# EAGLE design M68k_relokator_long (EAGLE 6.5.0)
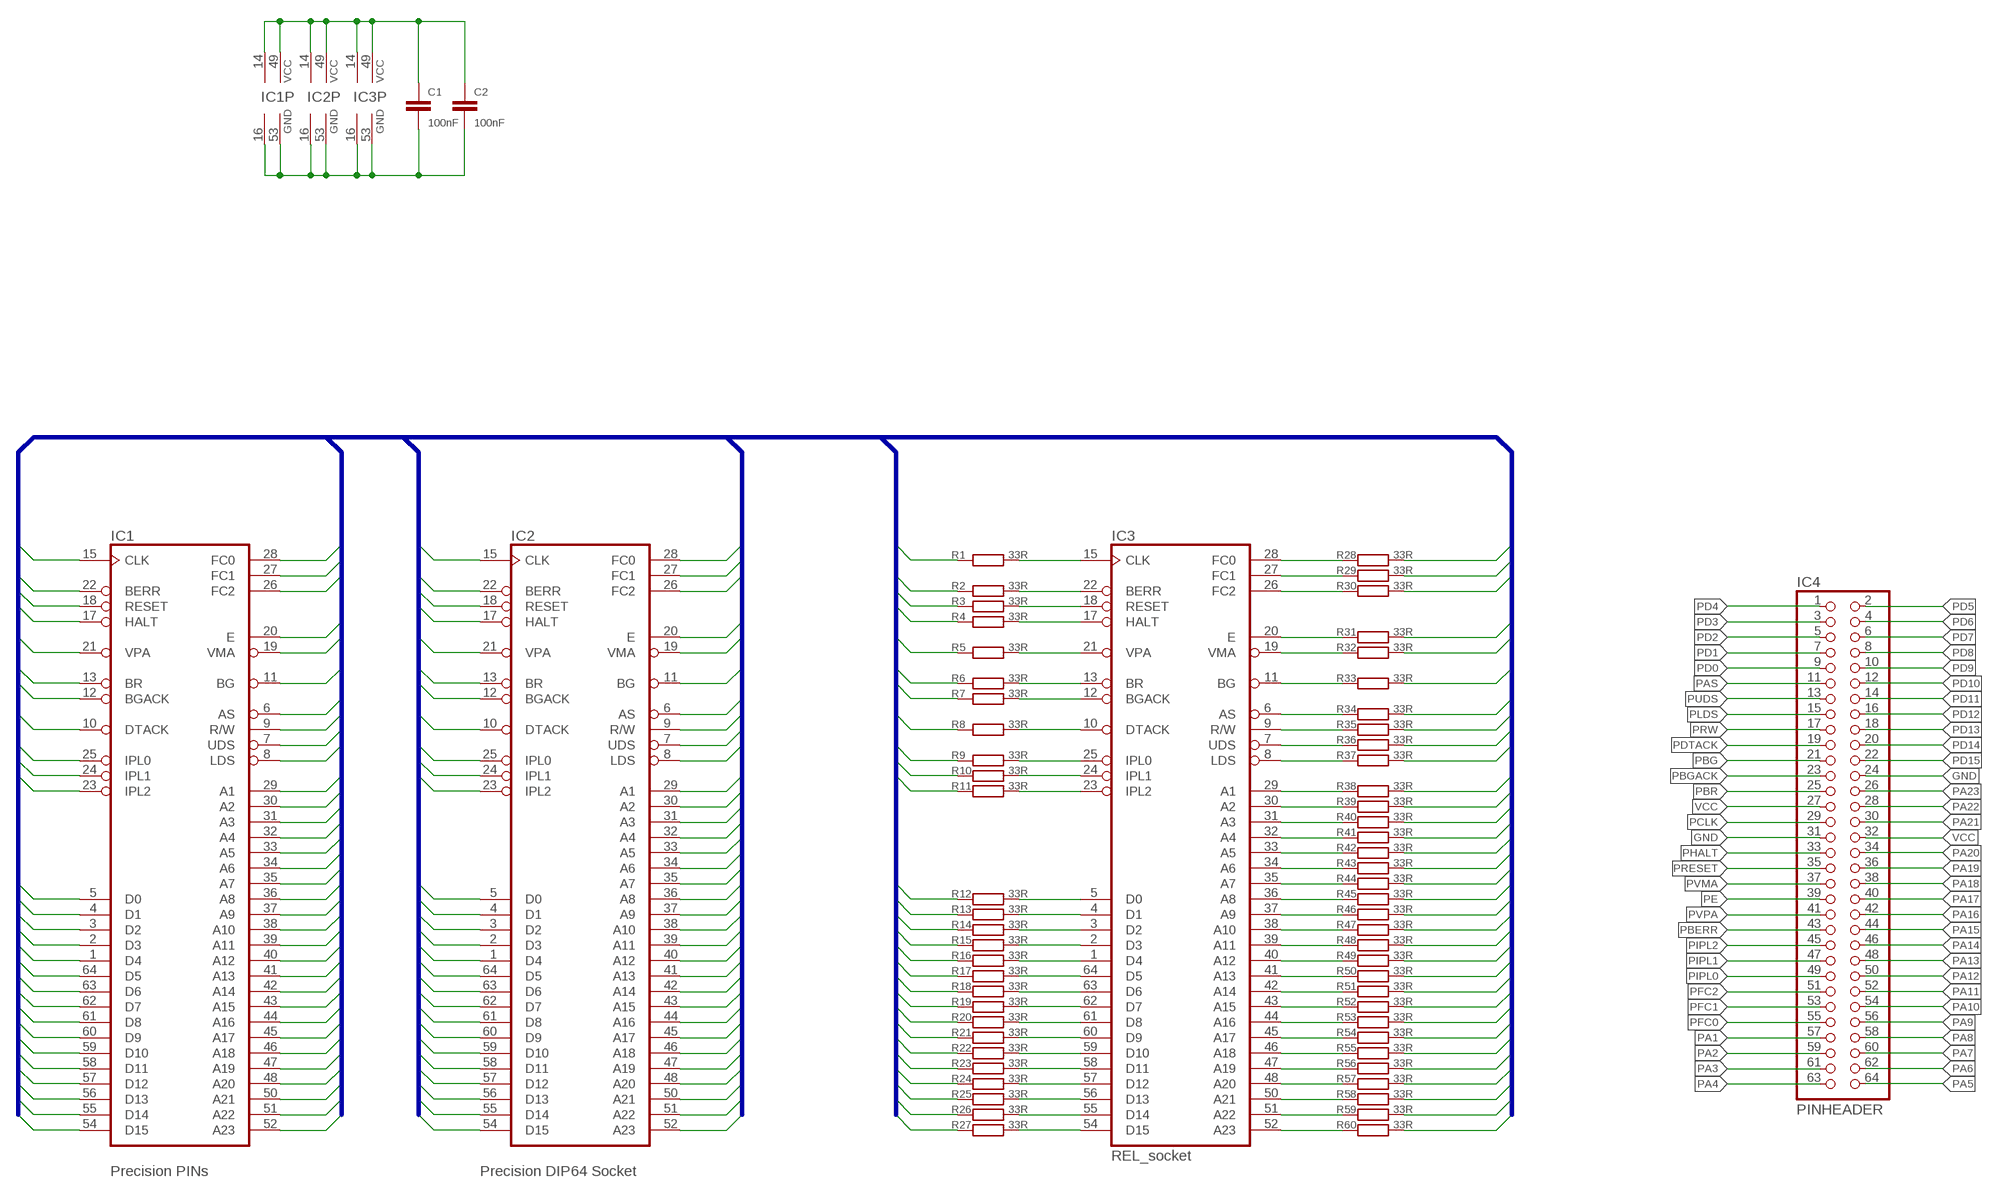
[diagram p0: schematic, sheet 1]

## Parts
C1  100nF  C-EUC0805  [C0805]
C2  100nF  C-EUC0805  [C0805]
IC1  Precision PINs  MC68000P  [DIL64]
IC2  Precision DIP64 Socket  MC68000P  [DIL64]
IC3  REL_socket  MC68000P  [DIL64]
IC4  PINHEADER  PINHD-2X32  [2X32]
R1  33R  R-EU_R0805  [R0805]
R2  33R  R-EU_R0805  [R0805]
R3  33R  R-EU_R0805  [R0805]
R4  33R  R-EU_R0805  [R0805]
R5  33R  R-EU_R0805  [R0805]
R6  33R  R-EU_R0805  [R0805]
R7  33R  R-EU_R0805  [R0805]
R8  33R  R-EU_R0805  [R0805]
R9  33R  R-EU_R0805  [R0805]
R10  33R  R-EU_R0805  [R0805]
R11  33R  R-EU_R0805  [R0805]
R12  33R  R-EU_R0805  [R0805]
R13  33R  R-EU_R0805  [R0805]
R14  33R  R-EU_R0805  [R0805]
R15  33R  R-EU_R0805  [R0805]
R16  33R  R-EU_R0805  [R0805]
R17  33R  R-EU_R0805  [R0805]
R18  33R  R-EU_R0805  [R0805]
R19  33R  R-EU_R0805  [R0805]
R20  33R  R-EU_R0805  [R0805]
R21  33R  R-EU_R0805  [R0805]
R22  33R  R-EU_R0805  [R0805]
R23  33R  R-EU_R0805  [R0805]
R24  33R  R-EU_R0805  [R0805]
R25  33R  R-EU_R0805  [R0805]
R26  33R  R-EU_R0805  [R0805]
R27  33R  R-EU_R0805  [R0805]
R28  33R  R-EU_R0805  [R0805]
R29  33R  R-EU_R0805  [R0805]
R30  33R  R-EU_R0805  [R0805]
R31  33R  R-EU_R0805  [R0805]
R32  33R  R-EU_R0805  [R0805]
R33  33R  R-EU_R0805  [R0805]
R34  33R  R-EU_R0805  [R0805]
R35  33R  R-EU_R0805  [R0805]
R36  33R  R-EU_R0805  [R0805]
R37  33R  R-EU_R0805  [R0805]
R38  33R  R-EU_R0805  [R0805]
R39  33R  R-EU_R0805  [R0805]
R40  33R  R-EU_R0805  [R0805]
R41  33R  R-EU_R0805  [R0805]
R42  33R  R-EU_R0805  [R0805]
R43  33R  R-EU_R0805  [R0805]
R44  33R  R-EU_R0805  [R0805]
R45  33R  R-EU_R0805  [R0805]
R46  33R  R-EU_R0805  [R0805]
R47  33R  R-EU_R0805  [R0805]
R48  33R  R-EU_R0805  [R0805]
R49  33R  R-EU_R0805  [R0805]
R50  33R  R-EU_R0805  [R0805]
R51  33R  R-EU_R0805  [R0805]
R52  33R  R-EU_R0805  [R0805]
R53  33R  R-EU_R0805  [R0805]
R54  33R  R-EU_R0805  [R0805]
R55  33R  R-EU_R0805  [R0805]
R56  33R  R-EU_R0805  [R0805]
R57  33R  R-EU_R0805  [R0805]
R58  33R  R-EU_R0805  [R0805]
R59  33R  R-EU_R0805  [R0805]
R60  33R  R-EU_R0805  [R0805]

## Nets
A1: IC1.29(A1) IC2.29(A1) R38.2
A2: IC1.30(A2) IC2.30(A2) R39.2
A3: IC1.31(A3) IC2.31(A3) R40.2
A4: IC1.32(A4) IC2.32(A4) R41.2
A5: IC1.33(A5) IC2.33(A5) R42.2
A6: IC1.34(A6) IC2.34(A6) R43.2
A7: IC1.35(A7) IC2.35(A7) R44.2
A8: IC1.36(A8) IC2.36(A8) R45.2
A9: IC1.37(A9) IC2.37(A9) R46.2
A10: IC1.38(A10) IC2.38(A10) R47.2
A11: IC1.39(A11) IC2.39(A11) R48.2
A12: IC1.40(A12) IC2.40(A12) R49.2
A13: IC1.41(A13) IC2.41(A13) R50.2
A14: IC1.42(A14) IC2.42(A14) R51.2
A15: IC1.43(A15) IC2.43(A15) R52.2
A16: IC1.44(A16) IC2.44(A16) R53.2
A17: IC1.45(A17) IC2.45(A17) R54.2
A18: IC1.46(A18) IC2.46(A18) R55.2
A19: IC1.47(A19) IC2.47(A19) R56.2
A20: IC1.48(A20) IC2.48(A20) R57.2
A21: IC1.50(A21) IC2.50(A21) R58.2
A22: IC1.51(A22) IC2.51(A22) R59.2
A23: IC1.52(A23) IC2.52(A23) R60.2
AS: IC1.6(AS) IC2.6(AS) R34.2
BERR: IC1.22(BERR) IC2.22(BERR) R2.1
BG: IC1.11(BG) IC2.11(BG) R33.2
BGACK: IC1.12(BGACK) IC2.12(BGACK) R7.1
BR: IC1.13(BR) IC2.13(BR) R6.1
CLK: IC1.15(CLK) IC2.15(CLK) R1.1
D0: IC1.5(D0) IC2.5(D0) R12.1
D1: IC1.4(D1) IC2.4(D1) R13.1
D2: IC1.3(D2) IC2.3(D2) R14.1
D3: IC1.2(D3) IC2.2(D3) R15.1
D4: IC1.1(D4) IC2.1(D4) R16.1
D5: IC1.64(D5) IC2.64(D5) R17.1
D6: IC1.63(D6) IC2.63(D6) R18.1
D7: IC1.62(D7) IC2.62(D7) R19.1
D8: IC1.61(D8) IC2.61(D8) R20.1
D9: IC1.60(D9) IC2.60(D9) R21.1
D10: IC1.59(D10) IC2.59(D10) R22.1
D11: IC1.58(D11) IC2.58(D11) R23.1
D12: IC1.57(D12) IC2.57(D12) R24.1
D13: IC1.56(D13) IC2.56(D13) R25.1
D14: IC1.55(D14) IC2.55(D14) R26.1
D15: IC1.54(D15) IC2.54(D15) R27.1
DTACK: IC1.10(DTACK) IC2.10(DTACK) R8.1
E: IC1.20(E) IC2.20(E) R31.2
FC0: IC1.28(FC0) IC2.28(FC0) R28.2
FC1: IC1.27(FC1) IC2.27(FC1) R29.2
FC2: IC1.26(FC2) IC2.26(FC2) R30.2
GND: C1.2 C2.2 IC1.16(GND) IC1.53(GND) IC2.16(GND) IC2.53(GND) IC3.16(GND) IC3.53(GND) IC4.24 IC4.31
HALT: IC1.17(HALT) IC2.17(HALT) R4.1
IPL0: IC1.25(IPL0) IC2.25(IPL0) R9.1
IPL1: IC1.24(IPL1) IC2.24(IPL1) R10.1
IPL2: IC1.23(IPL2) IC2.23(IPL2) R11.1
LDS: IC1.8(LDS) IC2.8(LDS) R37.2
PA1: IC3.29(A1) IC4.57 R38.1
PA2: IC3.30(A2) IC4.59 R39.1
PA3: IC3.31(A3) IC4.61 R40.1
PA4: IC3.32(A4) IC4.63 R41.1
PA5: IC3.33(A5) IC4.64 R42.1
PA6: IC3.34(A6) IC4.62 R43.1
PA7: IC3.35(A7) IC4.60 R44.1
PA8: IC3.36(A8) IC4.58 R45.1
PA9: IC3.37(A9) IC4.56 R46.1
PA10: IC3.38(A10) IC4.54 R47.1
PA11: IC3.39(A11) IC4.52 R48.1
PA12: IC3.40(A12) IC4.50 R49.1
PA13: IC3.41(A13) IC4.48 R50.1
PA14: IC3.42(A14) IC4.46 R51.1
PA15: IC3.43(A15) IC4.44 R52.1
PA16: IC3.44(A16) IC4.42 R53.1
PA17: IC3.45(A17) IC4.40 R54.1
PA18: IC3.46(A18) IC4.38 R55.1
PA19: IC3.47(A19) IC4.36 R56.1
PA20: IC3.48(A20) IC4.34 R57.1
PA21: IC3.50(A21) IC4.30 R58.1
PA22: IC3.51(A22) IC4.28 R59.1
PA23: IC3.52(A23) IC4.26 R60.1
PAS: IC3.6(AS) IC4.11 R34.1
PBERR: IC3.22(BERR) IC4.43 R2.2
PBG: IC3.11(BG) IC4.21 R33.1
PBGACK: IC3.12(BGACK) IC4.23 R7.2
PBR: IC3.13(BR) IC4.25 R6.2
PCLK: IC3.15(CLK) IC4.29 R1.2
PD0: IC3.5(D0) IC4.9 R12.2
PD1: IC3.4(D1) IC4.7 R13.2
PD2: IC3.3(D2) IC4.5 R14.2
PD3: IC3.2(D3) IC4.3 R15.2
PD4: IC3.1(D4) IC4.1 R16.2
PD5: IC3.64(D5) IC4.2 R17.2
PD6: IC3.63(D6) IC4.4 R18.2
PD7: IC3.62(D7) IC4.6 R19.2
PD8: IC3.61(D8) IC4.8 R20.2
PD9: IC3.60(D9) IC4.10 R21.2
PD10: IC3.59(D10) IC4.12 R22.2
PD11: IC3.58(D11) IC4.14 R23.2
PD12: IC3.57(D12) IC4.16 R24.2
PD13: IC3.56(D13) IC4.18 R25.2
PD14: IC3.55(D14) IC4.20 R26.2
PD15: IC3.54(D15) IC4.22 R27.2
PDTACK: IC3.10(DTACK) IC4.19 R8.2
PE: IC3.20(E) IC4.39 R31.1
PFC0: IC3.28(FC0) IC4.55 R28.1
PFC1: IC3.27(FC1) IC4.53 R29.1
PFC2: IC3.26(FC2) IC4.51 R30.1
PHALT: IC3.17(HALT) IC4.33 R4.2
PIPL0: IC3.25(IPL0) IC4.49 R9.2
PIPL1: IC3.24(IPL1) IC4.47 R10.2
PIPL2: IC3.23(IPL2) IC4.45 R11.2
PLDS: IC3.8(LDS) IC4.15 R37.1
PRESET: IC3.18(RESET) IC4.35 R3.2
PRW: IC3.9(R/W) IC4.17 R35.1
PUDS: IC3.7(UDS) IC4.13 R36.1
PVMA: IC3.19(VMA) IC4.37 R32.1
PVPA: IC3.21(VPA) IC4.41 R5.2
RESET: IC1.18(RESET) IC2.18(RESET) R3.1
RW: IC1.9(R/W) IC2.9(R/W) R35.2
UDS: IC1.7(UDS) IC2.7(UDS) R36.2
VCC: C1.1 C2.1 IC1.14(VCC) IC1.49(VCC) IC2.14(VCC) IC2.49(VCC) IC3.14(VCC) IC3.49(VCC) IC4.27 IC4.32
VMA: IC1.19(VMA) IC2.19(VMA) R32.2
VPA: IC1.21(VPA) IC2.21(VPA) R5.1

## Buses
D[0..15],IPL[0..2],DTACK,BGACK,BR,VPA,HALT,RESET,BERR,CLK,FC[0..2],E,VMA,BG,AS,RW,UDS,LDS,A[1..23]

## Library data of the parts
C1 C2 = rcl:C-EU: CAPACITOR, European symbol
IC1-IC3 = micro-mc68000:MC68000P: 68xxx PROCESSOR; OC_FARNELL: unknown; OC_NEWARK: unknown
IC4 = pinhead:PINHD-2X32
R1-R60 = rcl:R-EU_: RESISTOR, European symbol

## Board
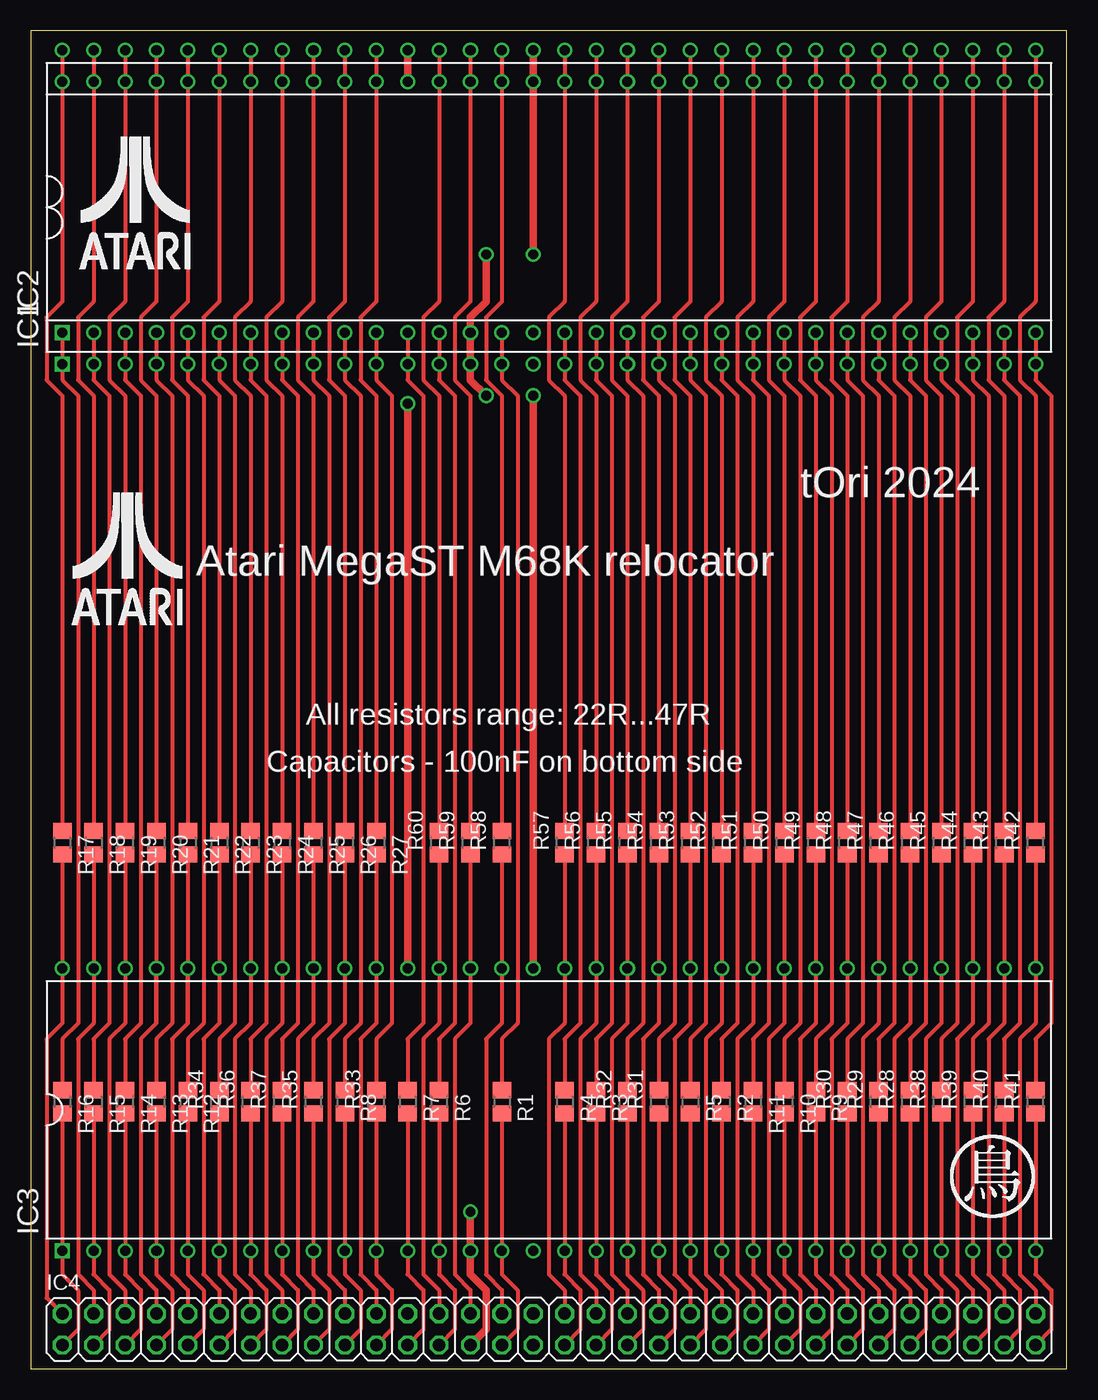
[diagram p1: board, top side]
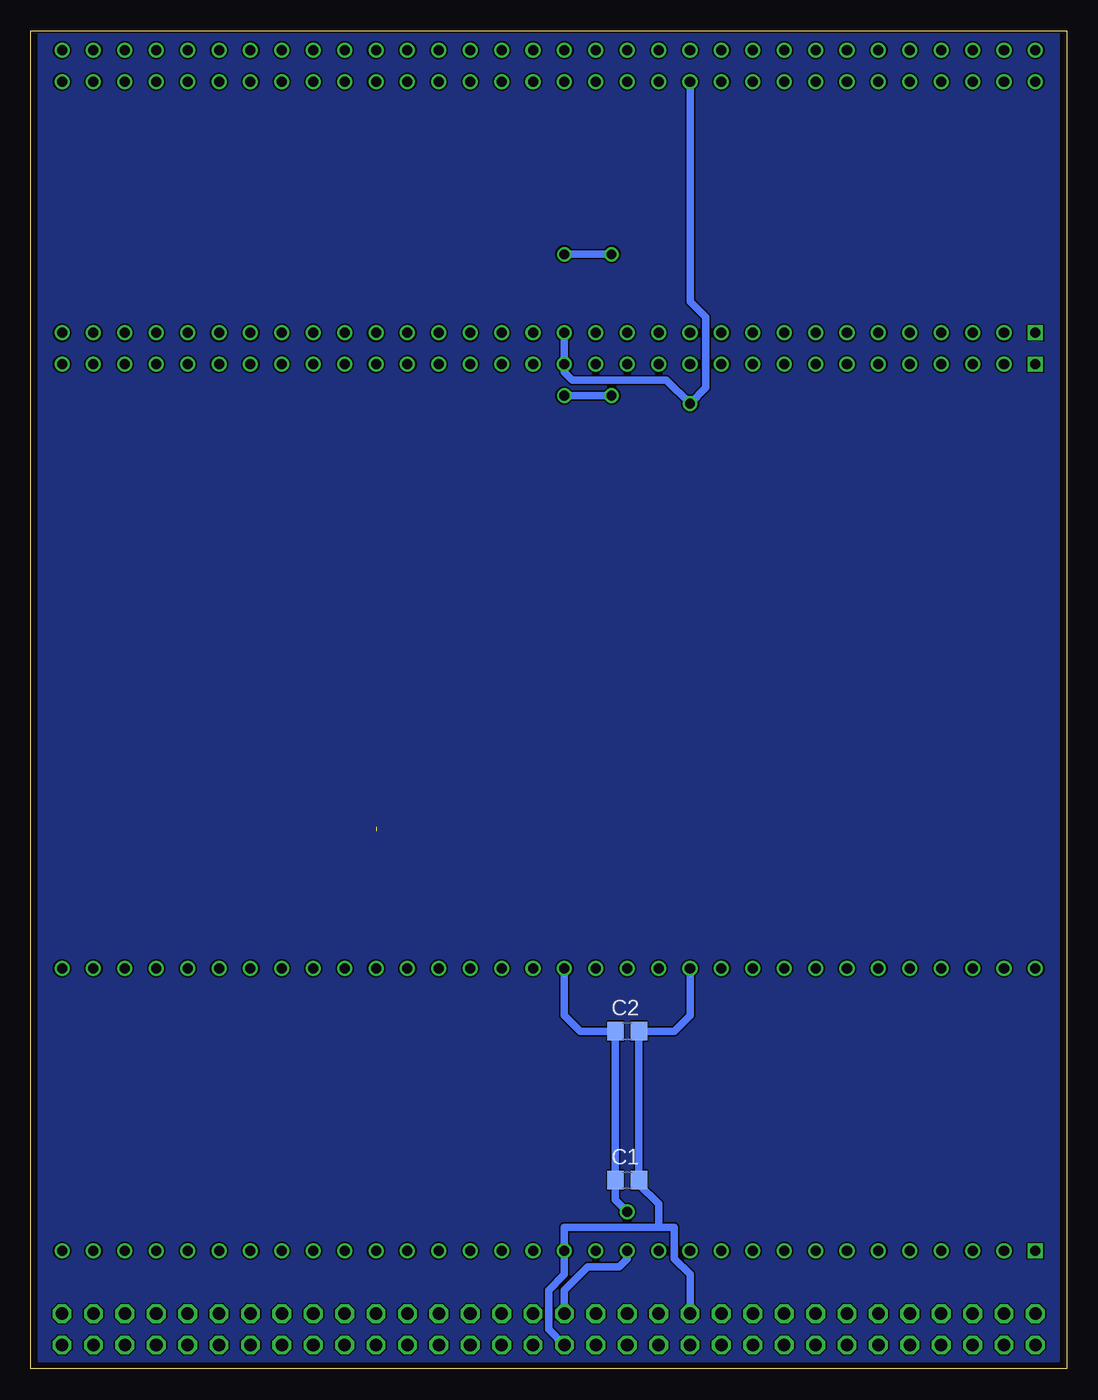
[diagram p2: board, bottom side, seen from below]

Size 83.8 x 108.26 mm. Coordinates in mm from the lower left corner, seen from the top.
Outline: 0,0 83.8,0 83.8,108.26 0,108.26 0,0
Copper layers (1*16): Top 0.035mm / dielectric 0.2mm / Bottom 0.035mm
Design rules "jlcpcb-2-layer": minimum track width 3.5mil, minimum drill 0.2mm, track to track 5mil, track to pad 5mil, pad to pad 5mil, via to via 5mil, smd to smd 0mil, copper to edge 0.1mm, drill to drill 5mil, minimum pad ring 4mil, minimum via ring 4mil, stop-mask expansion 3mil, vias tented up to drill 100mil, thermal gap 10mil

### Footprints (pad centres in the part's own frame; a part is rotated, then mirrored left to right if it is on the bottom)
C0805 = smd 1.3 x 1.5: 1 -0.95,0; 2 0.95,0
DIL64 = drill 0.813 square: 1 -39.37,-11.43 | drill 0.813: 2 -36.83,-11.43; 3 -34.29,-11.43; 4 -31.75,-11.43; 5 -29.21,-11.43; 6 -26.67,-11.43; 7 -24.13,-11.43; 8 -21.59,-11.43; 9 -19.05,-11.43; 10 -16.51,-11.43; 11 -13.97,-11.43; 12 -11.43,-11.43; 13 -8.89,-11.43; 14 -6.35,-11.43; 15 -3.81,-11.43; 16 -1.27,-11.43; 17 1.27,-11.43; 18 3.81,-11.43; 19 6.35,-11.43; 20 8.89,-11.43; 21 11.43,-11.43; 22 13.97,-11.43; 23 16.51,-11.43; 24 19.05,-11.43; 25 21.59,-11.43; 26 24.13,-11.43; 27 26.67,-11.43; 28 29.21,-11.43; 29 31.75,-11.43; 30 34.29,-11.43; 31 36.83,-11.43; 32 39.37,-11.43; 33 39.37,11.43; 34 36.83,11.43; 35 34.29,11.43; 36 31.75,11.43; 37 29.21,11.43; 38 26.67,11.43; 39 24.13,11.43; 40 21.59,11.43; 41 19.05,11.43; 42 16.51,11.43; 43 13.97,11.43; 44 11.43,11.43; 45 8.89,11.43; 46 6.35,11.43; 47 3.81,11.43; 48 1.27,11.43; 49 -1.27,11.43; 50 -3.81,11.43; 51 -6.35,11.43; 52 -8.89,11.43; 53 -11.43,11.43; 54 -13.97,11.43; 55 -16.51,11.43; 56 -19.05,11.43; 57 -21.59,11.43; 58 -24.13,11.43; 59 -26.67,11.43; 60 -29.21,11.43; 61 -31.75,11.43; 62 -34.29,11.43; 63 -36.83,11.43; 64 -39.37,11.43
2X32 = drill 1.016 octagon: 1 -36.83,-1.27; 2 -36.83,1.27; 3 -34.29,-1.27; 4 -34.29,1.27; 5 -31.75,-1.27; 6 -31.75,1.27; 7 -29.21,-1.27; 8 -29.21,1.27; 9 -26.67,-1.27; 10 -26.67,1.27; 11 -24.13,-1.27; 12 -24.13,1.27; 13 -21.59,-1.27; 14 -21.59,1.27; 15 -19.05,-1.27; 16 -19.05,1.27; 17 -16.51,-1.27; 18 -16.51,1.27; 19 -13.97,-1.27; 20 -13.97,1.27; 21 -11.43,-1.27; 22 -11.43,1.27; 23 -8.89,-1.27; 24 -8.89,1.27; 25 -6.35,-1.27; 26 -6.35,1.27; 27 -3.81,-1.27; 28 -3.81,1.27; 29 -1.27,-1.27; 30 -1.27,1.27; 31 1.27,-1.27; 32 1.27,1.27; 33 3.81,-1.27; 34 3.81,1.27; 35 6.35,-1.27; 36 6.35,1.27; 37 8.89,-1.27; 38 8.89,1.27; 39 11.43,-1.27; 40 11.43,1.27; 41 13.97,-1.27; 42 13.97,1.27; 43 16.51,-1.27; 44 16.51,1.27; 45 19.05,-1.27; 46 19.05,1.27; 47 21.59,-1.27; 48 21.59,1.27; 49 24.13,-1.27; 50 24.13,1.27; 51 26.67,-1.27; 52 26.67,1.27; 53 29.21,-1.27; 54 29.21,1.27; 55 31.75,-1.27; 56 31.75,1.27; 57 34.29,-1.27; 58 34.29,1.27; 59 36.83,-1.27; 60 36.83,1.27; 61 39.37,-1.27; 62 39.37,1.27; 63 41.91,-1.27; 64 41.91,1.27
R0805 = smd 1.3 x 1.5: 1 -0.95,0; 2 0.95,0

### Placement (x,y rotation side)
C1  35.56,15.24 0 bottom
C2  35.56,27.31 0 bottom
IC1  41.91,92.71 0 top
IC2  41.91,95.25 0 top
IC3  41.91,20.96 0 top
IC4  39.37,3.18 0 top
R1  38.1,21.59 270 top
R2  55.88,21.59 270 top
R3  45.72,21.59 270 top
R4  43.18,21.59 270 top
R5  53.34,21.59 270 top
R6  33.02,21.59 270 top
R7  30.48,21.59 270 top
R8  25.4,21.59 270 top
R9  63.5,21.59 270 top
R10  60.96,21.59 270 top
R11  58.42,21.59 270 top
R12  12.7,21.59 270 top
R13  10.16,21.59 270 top
R14  7.62,21.59 270 top
R15  5.08,21.59 270 top
R16  2.54,21.59 270 top
R17  2.54,42.55 270 top
R18  5.08,42.55 270 top
R19  7.62,42.55 270 top
R20  10.16,42.55 270 top
R21  12.7,42.55 270 top
R22  15.24,42.55 270 top
R23  17.78,42.55 270 top
R24  20.32,42.55 270 top
R25  22.86,42.55 270 top
R26  25.4,42.55 270 top
R27  27.94,42.55 270 top
R28  71.12,21.59 90 top
R29  68.58,21.59 90 top
R30  66.04,21.59 90 top
R31  50.8,21.59 90 top
R32  48.26,21.59 90 top
R33  27.94,21.59 90 top
R34  15.24,21.59 90 top
R35  22.86,21.59 90 top
R36  17.78,21.59 90 top
R37  20.32,21.59 90 top
R38  73.66,21.59 90 top
R39  76.2,21.59 90 top
R40  78.74,21.59 90 top
R41  81.28,21.59 90 top
R42  81.28,42.55 90 top
R43  78.74,42.55 90 top
R44  76.2,42.55 90 top
R45  73.66,42.55 90 top
R46  71.12,42.55 90 top
R47  68.58,42.55 90 top
R48  66.04,42.55 90 top
R49  63.5,42.55 90 top
R50  60.96,42.55 90 top
R51  58.42,42.55 90 top
R52  55.88,42.55 90 top
R53  53.34,42.55 90 top
R54  50.8,42.55 90 top
R55  48.26,42.55 90 top
R56  45.72,42.55 90 top
R57  43.18,42.55 90 top
R58  38.1,42.55 90 top
R59  35.56,42.55 90 top
R60  33.02,42.55 90 top

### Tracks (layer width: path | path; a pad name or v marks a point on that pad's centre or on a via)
A1
  Top 0.305: IC2.29 IC1.29 73.66,80.01 74.93,78.74 74.93,27.94 73.66,26.67 R38.2
A2
  Top 0.305: IC2.30 IC1.30 76.2,80.01 77.47,78.74 77.47,27.94 76.2,26.67 R39.2
A3
  Top 0.305: IC2.31 IC1.31 78.74,80.01 80.01,78.74 80.01,27.94 78.74,26.67 R40.2
A4
  Top 0.305: IC2.32 IC1.32 81.28,80.01 82.55,78.74 82.55,27.94 81.28,26.67 R41.2
A5
  Top 0.305: IC2.33 IC1.33 81.28,86.36 80.01,85.09 80.01,80.01 81.28,78.74 R42.2
A6
  Top 0.305: IC2.34 IC1.34 78.74,86.36 77.47,85.09 77.47,80.01 78.74,78.74 R43.2
A7
  Top 0.305: IC2.35 IC1.35 76.2,86.36 74.93,85.09 74.93,80.01 76.2,78.74 R44.2
A8
  Top 0.305: IC2.36 IC1.36 73.66,86.36 72.39,85.09 72.39,80.01 73.66,78.74 R45.2
A9
  Top 0.305: IC2.37 IC1.37 71.12,86.36 69.85,85.09 69.85,80.01 71.12,78.74 R46.2
A10
  Top 0.305: IC2.38 IC1.38 68.58,86.36 67.31,85.09 67.31,80.01 68.58,78.74 R47.2
A11
  Top 0.305: IC2.39 IC1.39 66.04,86.36 64.77,85.09 64.77,80.01 66.04,78.74 R48.2
A12
  Top 0.305: IC2.40 IC1.40 63.5,86.36 62.23,85.09 62.23,80.01 63.5,78.74 R49.2
A13
  Top 0.305: IC2.41 IC1.41 60.96,86.36 59.69,85.09 59.69,80.01 60.96,78.74 R50.2
A14
  Top 0.305: IC2.42 IC1.42 58.42,86.36 57.15,85.09 57.15,80.01 58.42,78.74 R51.2
A15  (1 unrouted)
  Top 0.305: IC2.43 IC1.43 55.88,86.36 54.61,85.09 54.61,80.01 55.88,78.74 55.88,43.82
A16
  Top 0.305: IC2.44 IC1.44 53.34,86.36 52.07,85.09 52.07,80.01 53.34,78.74 R53.2
A17
  Top 0.305: IC2.45 IC1.45 50.8,86.36 49.53,85.09 49.53,80.01 50.8,78.74 R54.2
A18
  Top 0.305: IC2.46 IC1.46 48.26,86.36 46.99,85.09 46.99,80.01 48.26,78.74 R55.2
A19
  Top 0.305: IC2.47 IC1.47 45.72,86.36 44.45,85.09 44.45,80.01 45.72,78.74 R56.2
A20
  Top 0.305: IC2.48 IC1.48 43.18,86.36 41.91,85.09 41.91,80.01 43.18,78.74 R57.2
A21
  Top 0.305: IC2.50 IC1.50 38.1,86.36 36.83,85.09 36.83,80.01 38.1,78.74 R58.2
A22
  Top 0.305: IC2.51 IC1.51 35.56,86.36 34.29,85.09 34.29,80.01 35.56,78.74 R59.2
A23
  Top 0.305: IC2.52 IC1.52 33.02,86.36 31.75,85.09 31.75,80.01 33.02,78.74 R60.2
AS
  Top 0.305: IC2.6 IC1.6 15.24,80.01 16.51,78.74 16.51,27.94 15.24,26.67 R34.2
BERR
  Top 0.305: IC2.22 IC1.22 55.88,80.01 57.15,78.74 57.15,27.94 55.88,26.67 R2.1
BG
  Top 0.305: IC2.11 IC1.11 27.94,80.01 29.21,78.74 29.21,27.94 27.94,26.67 R33.2
BGACK
  Top 0.305: IC2.12 IC1.12 30.48,80.01 31.75,78.74 31.75,27.94 30.48,26.67 R7.1
BR
  Top 0.305: IC2.13 IC1.13 33.02,80.01 34.29,78.74 34.29,27.94 33.02,26.67 R6.1
CLK
  Top 0.305: IC2.15 IC1.15 38.1,80.01 39.37,78.74 39.37,27.94 38.1,26.67 R1.1
D0
  Top 0.305: IC2.5 IC1.5 12.7,80.01 13.97,78.74 13.97,27.94 12.7,26.67 R12.1
D1
  Top 0.305: IC2.4 IC1.4 10.16,80.01 11.43,78.74 11.43,27.94 10.16,26.67 R13.1
D2
  Top 0.305: IC2.3 IC1.3 7.62,80.01 8.89,78.74 8.89,27.94 7.62,26.67 R14.1
D3
  Top 0.305: IC2.2 IC1.2 5.08,80.01 6.35,78.74 6.35,27.94 5.08,26.67 R15.1
D4
  Top 0.305: IC2.1 IC1.1 2.54,80.01 3.81,78.74 3.81,27.94 2.54,26.67 R16.1
D5
  Top 0.305: IC2.64 IC1.64 2.54,86.36 1.27,85.09 1.27,80.01 2.54,78.74 R17.1
D6
  Top 0.305: IC2.63 IC1.63 5.08,86.36 3.81,85.09 3.81,80.01 5.08,78.74 R18.1
D7
  Top 0.305: IC2.62 IC1.62 7.62,86.36 6.35,85.09 6.35,80.01 7.62,78.74 R19.1
D8
  Top 0.305: IC2.61 IC1.61 10.16,86.36 8.89,85.09 8.89,80.01 10.16,78.74 R20.1
D9
  Top 0.305: IC2.60 IC1.60 12.7,86.36 11.43,85.09 11.43,80.01 12.7,78.74 R21.1
D10
  Top 0.305: IC2.59 IC1.59 15.24,86.36 13.97,85.09 13.97,80.01 15.24,78.74 R22.1
D11
  Top 0.305: IC2.58 IC1.58 17.78,86.36 16.51,85.09 16.51,80.01 17.78,78.74 R23.1
D12
  Top 0.305: IC2.57 IC1.57 20.32,86.36 19.05,85.09 19.05,80.01 20.32,78.74 R24.1
D13
  Top 0.305: IC2.56 IC1.56 22.86,86.36 21.59,85.09 21.59,80.01 22.86,78.74 R25.1
D14
  Top 0.305: IC2.55 IC1.55 25.4,86.36 24.13,85.09 24.13,80.01 25.4,78.74 R26.1
D15
  Top 0.305: IC2.54 IC1.54 27.94,86.36 26.67,85.09 26.67,80.01 27.94,78.74 R27.1
DTACK
  Top 0.305: IC2.10 IC1.10 25.4,80.01 26.67,78.74 26.67,27.94 25.4,26.67 R8.1
E
  Top 0.305: IC2.20 IC1.20 50.8,80.01 52.07,78.74 52.07,27.94 50.8,26.67 R31.2
FC0
  Top 0.305: IC2.28 IC1.28 71.12,80.01 72.39,78.74 72.39,27.94 71.12,26.67 R28.2
FC1
  Top 0.305: IC2.27 IC1.27 68.58,80.01 69.85,78.74 69.85,27.94 68.58,26.67 R29.2
FC2
  Top 0.305: IC2.26 IC1.26 66.04,80.01 67.31,78.74 67.31,27.94 66.04,26.67 R30.2
GND  (via drill 0.8)
  Top 0.61: IC2.53 IC1.53 | v30.48,78.11 IC3.53
  Bottom 0.61: IC3.53 30.48,28.58 31.75,27.31 C2.2 C1.2 34.61,14.93 33.02,13.34 33.02,11.43 | 33.02,11.43 40.64,11.43 IC3.16 40.64,7.62 41.91,6.35 41.91,3.18 IC4.31 | IC4.24 30.48,7.62 31.75,8.89 31.75,11.43 33.02,11.43 | IC2.16 IC1.16 40.64,80.65 40.01,80.01 32.38,80.01 v30.48,78.11 29.21,79.38 29.21,85.09 30.48,86.36 IC1.53
HALT
  Top 0.305: IC2.17 IC1.17 43.18,80.01 44.45,78.74 44.45,27.94 43.18,26.67 R4.1
IPL0
  Top 0.305: IC2.25 IC1.25 63.5,80.01 64.77,78.74 64.77,27.94 63.5,26.67 R9.1
IPL1
  Top 0.305: IC2.24 IC1.24 60.96,80.01 62.23,78.74 62.23,27.94 60.96,26.67 R10.1
IPL2
  Top 0.305: IC2.23 IC1.23 58.42,80.01 59.69,78.74 59.69,27.94 58.42,26.67 R11.1
LDS
  Top 0.305: IC2.8 IC1.8 20.32,80.01 21.59,78.74 21.59,27.94 20.32,26.67 R37.2
N$1
  pour Bottom: 0.64,107.95 83.19,107.95 83.19,0.64 0.64,0.64
PA1
  Top 0.305: R38.1 IC3.29 73.66,7.62 74.93,6.35 74.93,3.18 IC4.57
PA2
  Top 0.305: R39.1 IC3.30 76.2,7.62 77.47,6.35 77.47,3.18 IC4.59
PA3
  Top 0.305: R40.1 IC3.31 78.74,7.62 80.01,6.35 80.01,3.18 IC4.61
PA4
  Top 0.305: R41.1 IC3.32 81.28,7.62 82.55,6.35 82.55,3.18 IC4.63
PA5
  Top 0.305: R42.1 IC3.33 81.28,27.94 80.01,26.67 80.01,7.62 81.28,6.35 IC4.64
PA6
  Top 0.305: R43.1 IC3.34 78.74,27.94 77.47,26.67 77.47,7.62 78.74,6.35 IC4.62
PA7
  Top 0.305: R44.1 IC3.35 76.2,27.94 74.93,26.67 74.93,7.62 76.2,6.35 IC4.60
PA8
  Top 0.305: R45.1 IC3.36 73.66,27.94 72.39,26.67 72.39,7.62 73.66,6.35 IC4.58
PA9
  Top 0.305: R46.1 IC3.37 71.12,27.94 69.85,26.67 69.85,7.62 71.12,6.35 IC4.56
PA10
  Top 0.305: R47.1 IC3.38 68.58,27.94 67.31,26.67 67.31,7.62 68.58,6.35 IC4.54
PA11
  Top 0.305: R48.1 IC3.39 66.04,27.94 64.77,26.67 64.77,7.62 66.04,6.35 IC4.52
PA12
  Top 0.305: R49.1 IC3.40 63.5,27.94 62.23,26.67 62.23,7.62 63.5,6.35 IC4.50
PA13
  Top 0.305: R50.1 IC3.41 60.96,27.94 59.69,26.67 59.69,7.62 60.96,6.35 IC4.48
PA14
  Top 0.305: R51.1 IC3.42 58.42,27.94 57.15,26.67 57.15,7.62 58.42,6.35 IC4.46
PA15
  Top 0.305: R52.1 IC3.43 55.88,27.94 54.61,26.67 54.61,7.62 55.88,6.35 IC4.44
PA16
  Top 0.305: R53.1 IC3.44 53.34,27.94 52.07,26.67 52.07,7.62 53.34,6.35 IC4.42
PA17
  Top 0.305: R54.1 IC3.45 50.8,27.94 49.53,26.67 49.53,7.62 50.8,6.35 IC4.40
PA18
  Top 0.305: R55.1 IC3.46 48.26,27.94 46.99,26.67 46.99,7.62 48.26,6.35 IC4.38
PA19
  Top 0.305: R56.1 IC3.47 45.72,27.94 44.45,26.67 44.45,7.62 45.72,6.35 IC4.36
PA20
  Top 0.305: R57.1 IC3.48 43.18,27.94 41.91,26.67 41.91,7.62 43.18,6.35 IC4.34
PA21
  Top 0.305: R58.1 IC3.50 38.1,27.94 36.83,26.67 36.83,7.62 38.1,6.35 IC4.30
PA22
  Top 0.305: R59.1 IC3.51 35.56,27.94 34.29,26.67 34.29,7.62 35.56,6.35 IC4.28
PA23
  Top 0.305: R60.1 IC3.52 33.02,27.94 31.75,26.67 31.75,7.62 33.02,6.35 IC4.26
PAS
  Top 0.305: R34.1 IC3.6 15.24,7.62 16.51,6.35 16.51,3.18 IC4.11
PBERR
  Top 0.305: R2.2 IC3.22 55.88,7.62 57.15,6.35 57.15,3.18 IC4.43
PBG
  Top 0.305: R33.1 IC3.11 27.94,7.62 29.21,6.35 29.21,3.18 IC4.21
PBGACK
  Top 0.305: R7.2 IC3.12 30.48,7.62 31.75,6.35 31.75,3.18 IC4.23
PBR
  Top 0.305: R6.2 IC3.13 33.02,7.62 34.29,6.35 34.29,3.18 IC4.25
PCLK
  Top 0.305: R1.2 IC3.15 38.1,7.62 39.37,6.35 39.37,3.18 IC4.29
PD0
  Top 0.305: R12.2 IC3.5 12.7,7.62 13.97,6.35 13.97,3.18 IC4.9
PD1
  Top 0.305: R13.2 IC3.4 10.16,7.62 11.43,6.35 11.43,3.18 IC4.7
PD2
  Top 0.305: R14.2 IC3.3 7.62,7.62 8.89,6.35 8.89,3.18 IC4.5
PD3
  Top 0.305: R15.2 IC3.2 5.08,7.62 6.35,6.35 6.35,3.18 IC4.3
PD4
  Top 0.305: R16.2 IC3.1 2.54,7.62 3.81,6.35 3.81,3.18 IC4.1
PD5
  Top 0.305: R17.2 IC3.64 2.54,27.94 1.27,26.67 1.27,5.72 IC4.2
PD6
  Top 0.305: R18.2 IC3.63 5.08,27.94 3.81,26.67 3.81,7.62 5.08,6.35 IC4.4
PD7
  Top 0.305: R19.2 IC3.62 7.62,27.94 6.35,26.67 6.35,7.62 7.62,6.35 IC4.6
PD8
  Top 0.305: R20.2 10.16,27.94 | 10.16,27.94 IC3.61 10.16,27.94 | 10.16,27.94 8.89,26.67 8.89,7.62 10.16,6.35 IC4.8
PD9
  Top 0.305: R21.2 12.7,27.94 | 12.7,27.94 IC3.60 12.7,27.94 | 12.7,27.94 11.43,26.67 11.43,7.62 12.7,6.35 IC4.10
PD10
  Top 0.305: R22.2 IC3.59 15.24,27.94 13.97,26.67 13.97,7.62 15.24,6.35 IC4.12
PD11
  Top 0.305: R23.2 IC3.58 17.78,27.94 16.51,26.67 16.51,7.62 17.78,6.35 IC4.14
PD12
  Top 0.305: R24.2 IC3.57 20.32,27.94 19.05,26.67 19.05,7.62 20.32,6.35 IC4.16
PD13
  Top 0.305: R25.2 IC3.56 22.86,27.94 21.59,26.67 21.59,7.62 22.86,6.35 IC4.18
PD14
  Top 0.305: R26.2 IC3.55 25.4,27.94 24.13,26.67 24.13,7.62 25.4,6.35 IC4.20
PD15
  Top 0.305: R27.2 IC3.54 27.94,27.94 26.67,26.67 26.67,7.62 27.94,6.35 IC4.22
PDTACK
  Top 0.305: R8.2 IC3.10 25.4,7.62 26.67,6.35 26.67,3.18 IC4.19
PE
  Top 0.305: R31.1 IC3.20 50.8,7.62 52.07,6.35 52.07,3.18 IC4.39
PFC0
  Top 0.305: R28.1 IC3.28 71.12,7.62 72.39,6.35 72.39,3.18 IC4.55
PFC1
  Top 0.305: R29.1 IC3.27 68.58,7.62 69.85,6.35 69.85,3.18 IC4.53
PFC2
  Top 0.305: R30.1 IC3.26 66.04,7.62 67.31,6.35 67.31,3.18 IC4.51
PHALT
  Top 0.305: R4.2 IC3.17 43.18,7.62 44.45,6.35 44.45,3.18 IC4.33
PIPL0
  Top 0.305: R9.2 IC3.25 63.5,7.62 64.77,6.35 64.77,3.18 IC4.49
PIPL1
  Top 0.305: R10.2 IC3.24 60.96,7.62 62.23,6.35 62.23,3.18 IC4.47
PIPL2
  Top 0.305: R11.2 IC3.23 58.42,7.62 59.69,6.35 59.69,3.18 IC4.45
PLDS
  Top 0.305: R37.1 IC3.8 20.32,7.62 21.59,6.35 21.59,3.18 IC4.15
PRESET
  Top 0.305: R3.2 IC3.18 45.72,7.62 46.99,6.35 46.99,3.18 IC4.35
PRW
  Top 0.305: R35.1 IC3.9 22.86,7.62 24.13,6.35 24.13,3.18 IC4.17
PUDS
  Top 0.305: R36.1 IC3.7 17.78,7.62 19.05,6.35 19.05,3.18 IC4.13
PVMA
  Top 0.305: R32.1 IC3.19 48.26,7.62 49.53,6.35 49.53,3.18 IC4.37
PVPA
  Top 0.305: R5.2 IC3.21 53.34,7.62 54.61,6.35 54.61,3.18 IC4.41
RESET
  Top 0.305: IC2.18 IC1.18 45.72,80.01 46.99,78.74 46.99,27.94 45.72,26.67 R3.1
RW
  Top 0.305: IC2.9 IC1.9 22.86,80.01 24.13,78.74 24.13,27.94 22.86,26.67 R35.2
UDS
  Top 0.305: IC2.7 IC1.7 17.78,80.01 19.05,78.74 19.05,27.94 17.78,26.67 R36.2
VCC  (via drill 0.8)
  Top 0.61: IC2.49 IC1.49 v40.64,90.17 | v36.83,90.17 36.83,86.36 35.56,85.09 IC2.14 IC1.14 35.56,80.01 v36.83,78.74 | v40.64,78.74 IC3.49 | v35.56,12.7 IC3.14 35.56,7.62 36.83,6.35 36.83,3.18 IC4.27
  Bottom 0.61: v40.64,90.17 v36.83,90.17 | v36.83,78.74 v40.64,78.74 | IC3.49 40.64,28.58 39.37,27.31 C2.1 36.51,13.65 | 36.51,13.65 C1.1 36.51,13.65 | 36.51,13.65 v35.56,12.7 | IC4.32 40.64,6.35 38.74,8.26 36.2,8.26 35.56,8.89 IC3.14
VMA
  Top 0.305: IC2.19 IC1.19 48.26,80.01 49.53,78.74 49.53,27.94 48.26,26.67 R32.2
VPA
  Top 0.305: IC2.21 IC1.21 53.34,80.01 54.61,78.74 54.61,27.94 53.34,26.67 R5.1

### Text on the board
tPlace: tOri 2024 | Atari MegaST M68K relocator | All resistors range: 22R...47R | Capacitors - 100nF on bottom side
